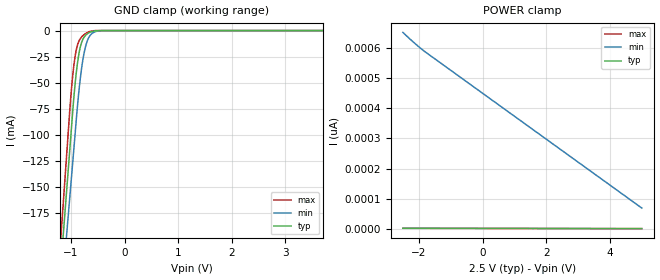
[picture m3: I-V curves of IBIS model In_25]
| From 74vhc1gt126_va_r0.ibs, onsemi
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|//////////////////////////////////////////////////////////////////////////////
|//////////////////////////////////////////////////////////////////////////////
[Model]  In_25
Model_type Input
Vinh =  1.00
Vinl =  0.28
|  variable   typ   min   max
C_comp   2.6pF   2.6pF   2.6pF
|//////////////////////////////////////////////////////////////////////////////
[Temperature Range]   25   125   -55
|//////////////////////////////////////////////////////////////////////////////
[Voltage Range]   2.50V   2.30V   2.70V
|//////////////////////////////////////////////////////////////////////////////
[POWER Clamp Reference] 2.50V   2.30V   2.70V
|//////////////////////////////////////////////////////////////////////////////
[GND Clamp Reference]   0V   0V   0V
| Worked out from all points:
|   GND clamp passes 1 mA (typ) near -0.61 V on its own axis
|//////////////////////////////////////////////////////////////////////////////
[GND Clamp]
|   Voltage   I(typ)   I(min)   I(max)
-2.5V     -1.111A    -1.066A    -1.164A
-1.18V    -222.1mA   -258.1mA   -193.9mA
-1.12V    -181.7mA   -221.4mA   -149.8mA
-1.08V    -154.7mA   -196.9mA   -120.4mA
-1V       -100.8mA   -147.9mA   -62.96mA
-920mV    -50.55mA   -98.9mA    -24.44mA
-860mV    -25.33mA   -63.27mA   -11.37mA
-800mV    -11.45mA   -36.21mA   -6.145mA
-740mV    -5.361mA   -18.26mA   -3.365mA
-680mV    -2.635mA   -8.098mA   -1.525mA
-400mV    -2.109uA   -41.44uA   -105nA
5V        1.982pA    655.9pA    1.732pA
|//////////////////////////////////////////////////////////////////////////////
[POWER Clamp]
|   Voltage   I(typ)   I(min)   I(max)
-2.5V     1.982pA    652pA      1.766pA
-2.16V    1.922pA    618.8pA    1.708pA
-1.82V    1.861pA    588.8pA    1.65pA
5V        645.8fA    68.84pA    483.6fA
